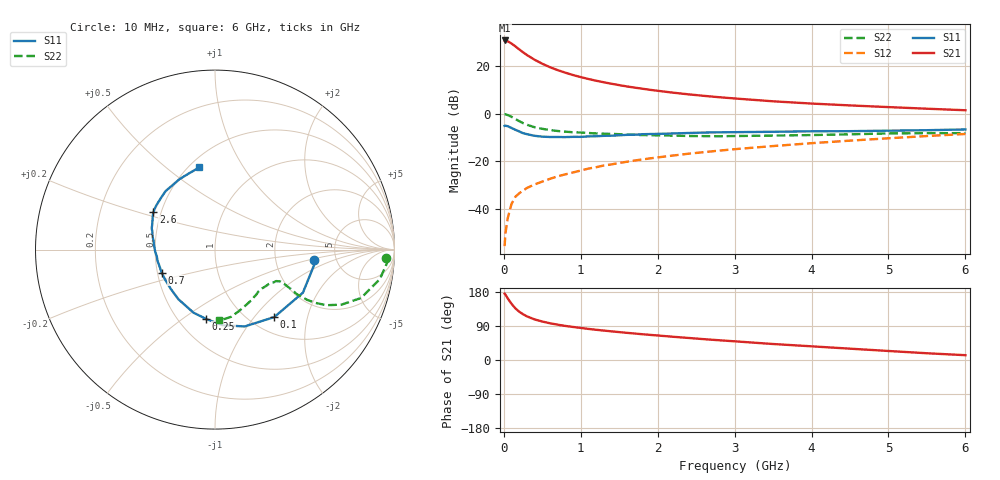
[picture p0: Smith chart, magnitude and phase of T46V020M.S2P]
! Infineon Technologies  Discrete & RF Semiconductors
! BFR182T
! Si NPN RF Bipolar Junction Transistor in SC75
! VCE = 6 V  IC = 20 mA
! Common Emitter S-Parameters:  October  1999
# GHz  S  MA  R  50
!  f  S11  S21  S12  S22
! GHz  MAG  ANG  MAG  ANG  MAG  ANG  MAG  ANG
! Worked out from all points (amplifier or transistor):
!   36 points, 10 MHz to 6 GHz, reference 50 ohm
!   highest |S21| = 30.6 dB at 10 MHz (marker M1)
!   |S21| within 3 dB of that: start of sweep to 171.1 MHz
!   unconditionally stable (mu >= 1): 744.9 MHz to 3.73 GHz
!   at 250 MHz: K = 0.62, MSG = 28.9 dB, |S12| = -32.2 dB
!   at 1.4 GHz: K = 1.09, MAG = 15.0 dB, |S12| = -21.2 dB
!   at 6 GHz: K = 0.85, MSG = 5.0 dB, |S12| = -8.5 dB
!   S11 on the Smith chart (normalised r, x): 10 MHz: 3.37, -0.57; 100 MHz: 1.27, -1.27; 250 MHz: 0.68, -0.62; 700 MHz: 0.53, -0.15; 2.6 GHz: 0.45, +0.23; 6 GHz: 0.56, +0.66
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0.01  0.553 -6.1  33.69 175.0  0.0017 76.0  0.9563 -2.7
0.02  0.5586 -9.0  33.46 172.8  0.0031 93.1  0.9633 -4.1
0.05  0.5454 -26.1  32.43 162.7  0.0065 84.9  0.9334 -10.1
0.1  0.5004 -48.7  29.04 148.3  0.013 74.6  0.8578 -18.3
0.15  0.4591 -68.9  25.34 136.3  0.0183 66.0  0.7687 -23.5
0.2  0.423 -84.5  21.95 127.5  0.0216 66.2  0.6945 -26.5
0.25  0.3897 -97.2  19.05 120.7  0.0246 63.1  0.6315 -28.0
0.3  0.3714 -108.8  16.73 115.2  0.0279 63.1  0.5856 -28.6
0.4  0.3436 -126.4  13.32 107.1  0.0331 64.0  0.5185 -28.6
0.5  0.3295 -138.7  10.99 101.5  0.038 65.2  0.4803 -27.5
0.6  0.3243 -148.6  9.304 96.9  0.0434 66.7  0.4532 -27.0
0.7  0.3239 -156.6  8.084 93.2  0.0489 67.8  0.4328 -26.5
0.9  0.3264 -168.8  6.378 87.2  0.0589 69.8  0.4071 -26.1
1.1  0.3337 -178.2  5.279 82.0  0.0709 70.3  0.3929 -26.7
1.3  0.3428 174.4  4.507 77.6  0.0824 70.5  0.3798 -27.9
1.6  0.3595 166.1  3.69 71.7  0.0986 70.3  0.3647 -30.1
2.2  0.3844 154.9  2.736 61.3  0.1331 69.5  0.3463 -36.8
2.6  0.4014 148.8  2.348 55.0  0.1565 68.3  0.3381 -41.8
3.5  0.4168 136.2  1.805 42.2  0.2098 64.6  0.3472 -54.4
4.5  0.4292 124.1  1.481 29.9  0.2722 59.5  0.3689 -69.4
5.5  0.4495 108.4  1.264 17.8  0.3397 53.6  0.3901 -82.0
6  0.4663 100.7  1.174 12.7  0.3753 50.0  0.3905 -87.1
